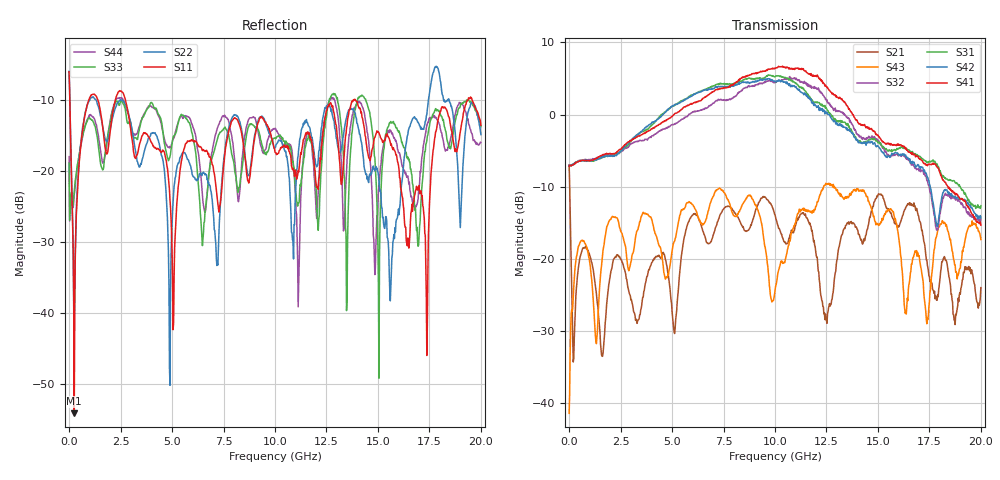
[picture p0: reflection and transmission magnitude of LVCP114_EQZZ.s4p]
!Agilent Technologies,N5230A,MY46400459,A.07.50.48
!Agilent N5230A: A.07.50.48
!Date: Monday, January 09, 2012 14:01:44
!Correction: S11(Full 4 Port(1,2,3,4))
!S12(Full 4 Port(1,2,3,4))
!S13(Full 4 Port(1,2,3,4))
!S14(Full 4 Port(1,2,3,4))
!S21(Full 4 Port(1,2,3,4))
!S22(Full 4 Port(1,2,3,4))
!S23(Full 4 Port(1,2,3,4))
!S24(Full 4 Port(1,2,3,4))
!S31(Full 4 Port(1,2,3,4))
!S32(Full 4 Port(1,2,3,4))
!S33(Full 4 Port(1,2,3,4))
!S34(Full 4 Port(1,2,3,4))
!S41(Full 4 Port(1,2,3,4))
!S42(Full 4 Port(1,2,3,4))
!S43(Full 4 Port(1,2,3,4))
!S44(Full 4 Port(1,2,3,4))
!S4P File: Measurements: <S11,S12,S13,S14>,
!<S21,S22,S23,S24>,
!<S31,S32,S33,S34>,
!<S41,S42,S43,S44>:
# Hz S  dB  R 50
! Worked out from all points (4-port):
!   801 points, 300 kHz to 20 GHz, reference 50 ohm
!   strongest paths, dB at 300 kHz, 5 GHz, 10 GHz, 15 GHz, 20 GHz:
!     S41: -7.2, -0.3, 6.4, -2.8, -15.3
!     S42: -7.1, 1.1, 4.6, -4.4, -14.3
!     S31: -7.1, 1.1, 5.2, -3.9, -12.6
!     S32: -7.0, -1.4, 4.4, -3.7, -14.5
!     S43: -41.4, -19.0, -24.4, -15.2, -17.3
!     S21: -7.0, -27.3, -13.9, -11.2, -24.0
!   lowest |S11| = -54.1 dB at 250.3 MHz (marker M1), VSWR 1.00, Z = 50.2 + j0.063 ohm
!   |S11| at or under -10 dB: 34.58 MHz to 948.9 MHz (914.3 MHz wide, 186 % of centre); 2.739 GHz to 13.8 GHz (11.06 GHz wide, 134 % of centre); 13.91 GHz to 19.37 GHz (5.454 GHz wide, 32.8 % of centre)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
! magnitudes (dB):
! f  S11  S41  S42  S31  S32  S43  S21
! 300 kHz  -6.0  -7.2  -7.1  -7.1  -7.0  -41.4  -7.0
! 250.3 MHz  -54.1  -6.9  -6.8  -6.9  -6.8  -22.8  -31.1
! 1.15 GHz  -9.1  -6.3  -6.3  -6.5  -6.1  -24.8  -21.3
! 4.9 GHz  -24.1  -0.5  0.9  1.0  -1.6  -21.0  -24.2
! 8.025 GHz  -12.5  4.3  4.1  4.3  2.5  -14.1  -13.6
! 17.38 GHz  -45.9  -6.9  -8.5  -6.7  -9.1  -29.0  -20.2
! 20 GHz  -13.5  -15.3  -14.3  -12.6  -14.5  -17.3  -24.0
